(* Logix 5000 DataType export Banner_Discrete_Host_Out_Mirroring_Cfg; software revision 33.00 *)

TYPE Banner_Discrete_Host_Out_Mirroring_Cfg :
STRUCT
   Enable : SINT;   // 0=Disabled, 1=Enabled.
   Port_Selection : SINT;   // 0=Port 1
   Channel_Selection : SINT;   // 0=Discrete 1, 1=Discrete 2.
   Mirroring_Inversion : SINT;   // 0=Not Inverted, 1=Inverted.
   Mirroring_Polarity : SINT;   // 0=NPN Output, 1=PNP Output.
   Output_Type : SINT;   // 0=Output with Internal Pull Up / Down, 1=Output Open Collector, 2=Output Push Pull.
END_STRUCT
END_TYPE
